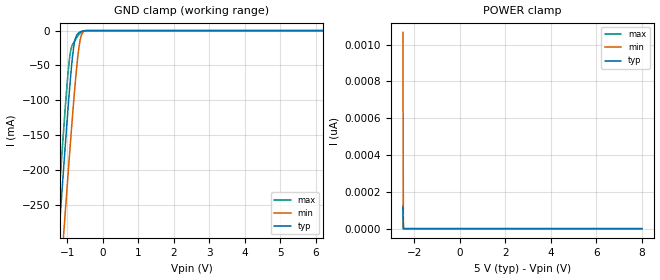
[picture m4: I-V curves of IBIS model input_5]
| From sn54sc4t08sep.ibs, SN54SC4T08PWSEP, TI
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|   input_5p0 Model
[Model]   input_5
Model_type   Input
Vinl = 0.85
Vinh = 2
|   typ   min   max
C_comp   3.5pF   3.4pF   3.7pF
[Voltage Range]   5   4.5   5.5
[Temperature Range]   25   125   -40
[Power Clamp Reference]   5   4.5   5.5
[GND Clamp Reference]   0   0   0
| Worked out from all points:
|   GND clamp passes 1 mA (typ) near -0.59 V on its own axis
[GND Clamp]
|   Voltage   I(typ)   I(min)   I(max)
-2.5V     -1.244A    -1.327A    -1.203A
-1.313V   -350.3mA   -444.6mA   -296.5mA
-1.23V    -289mA     -383.9mA   -234.5mA
-1.125V   -213.4mA   -308.8mA   -158.5mA
-1.072V   -176.4mA   -271.7mA   -121.6mA
-977.5mV  -111.7mA   -206mA     -60.6mA
-914.5mV  -71.44mA   -163.3mA   -31.85mA
-799mV    -17.49mA   -89.06mA   -15.38mA
-704.5mV  -4.594mA   -38.07mA   -7.858mA
-631mV    -1.797mA   -12.21mA   -3.542mA
-442mV    -17.94uA   -111.5uA   -18.13uA
8V        0A         0A         0A
[POWER Clamp]
|   Voltage   I(typ)   I(min)   I(max)
-2.5V     113.6pA    1.066nA    123.3pA
-2.479V   0A         0A         0A
-1mV      0A         0A         0A
8V        0A         0A         0A
